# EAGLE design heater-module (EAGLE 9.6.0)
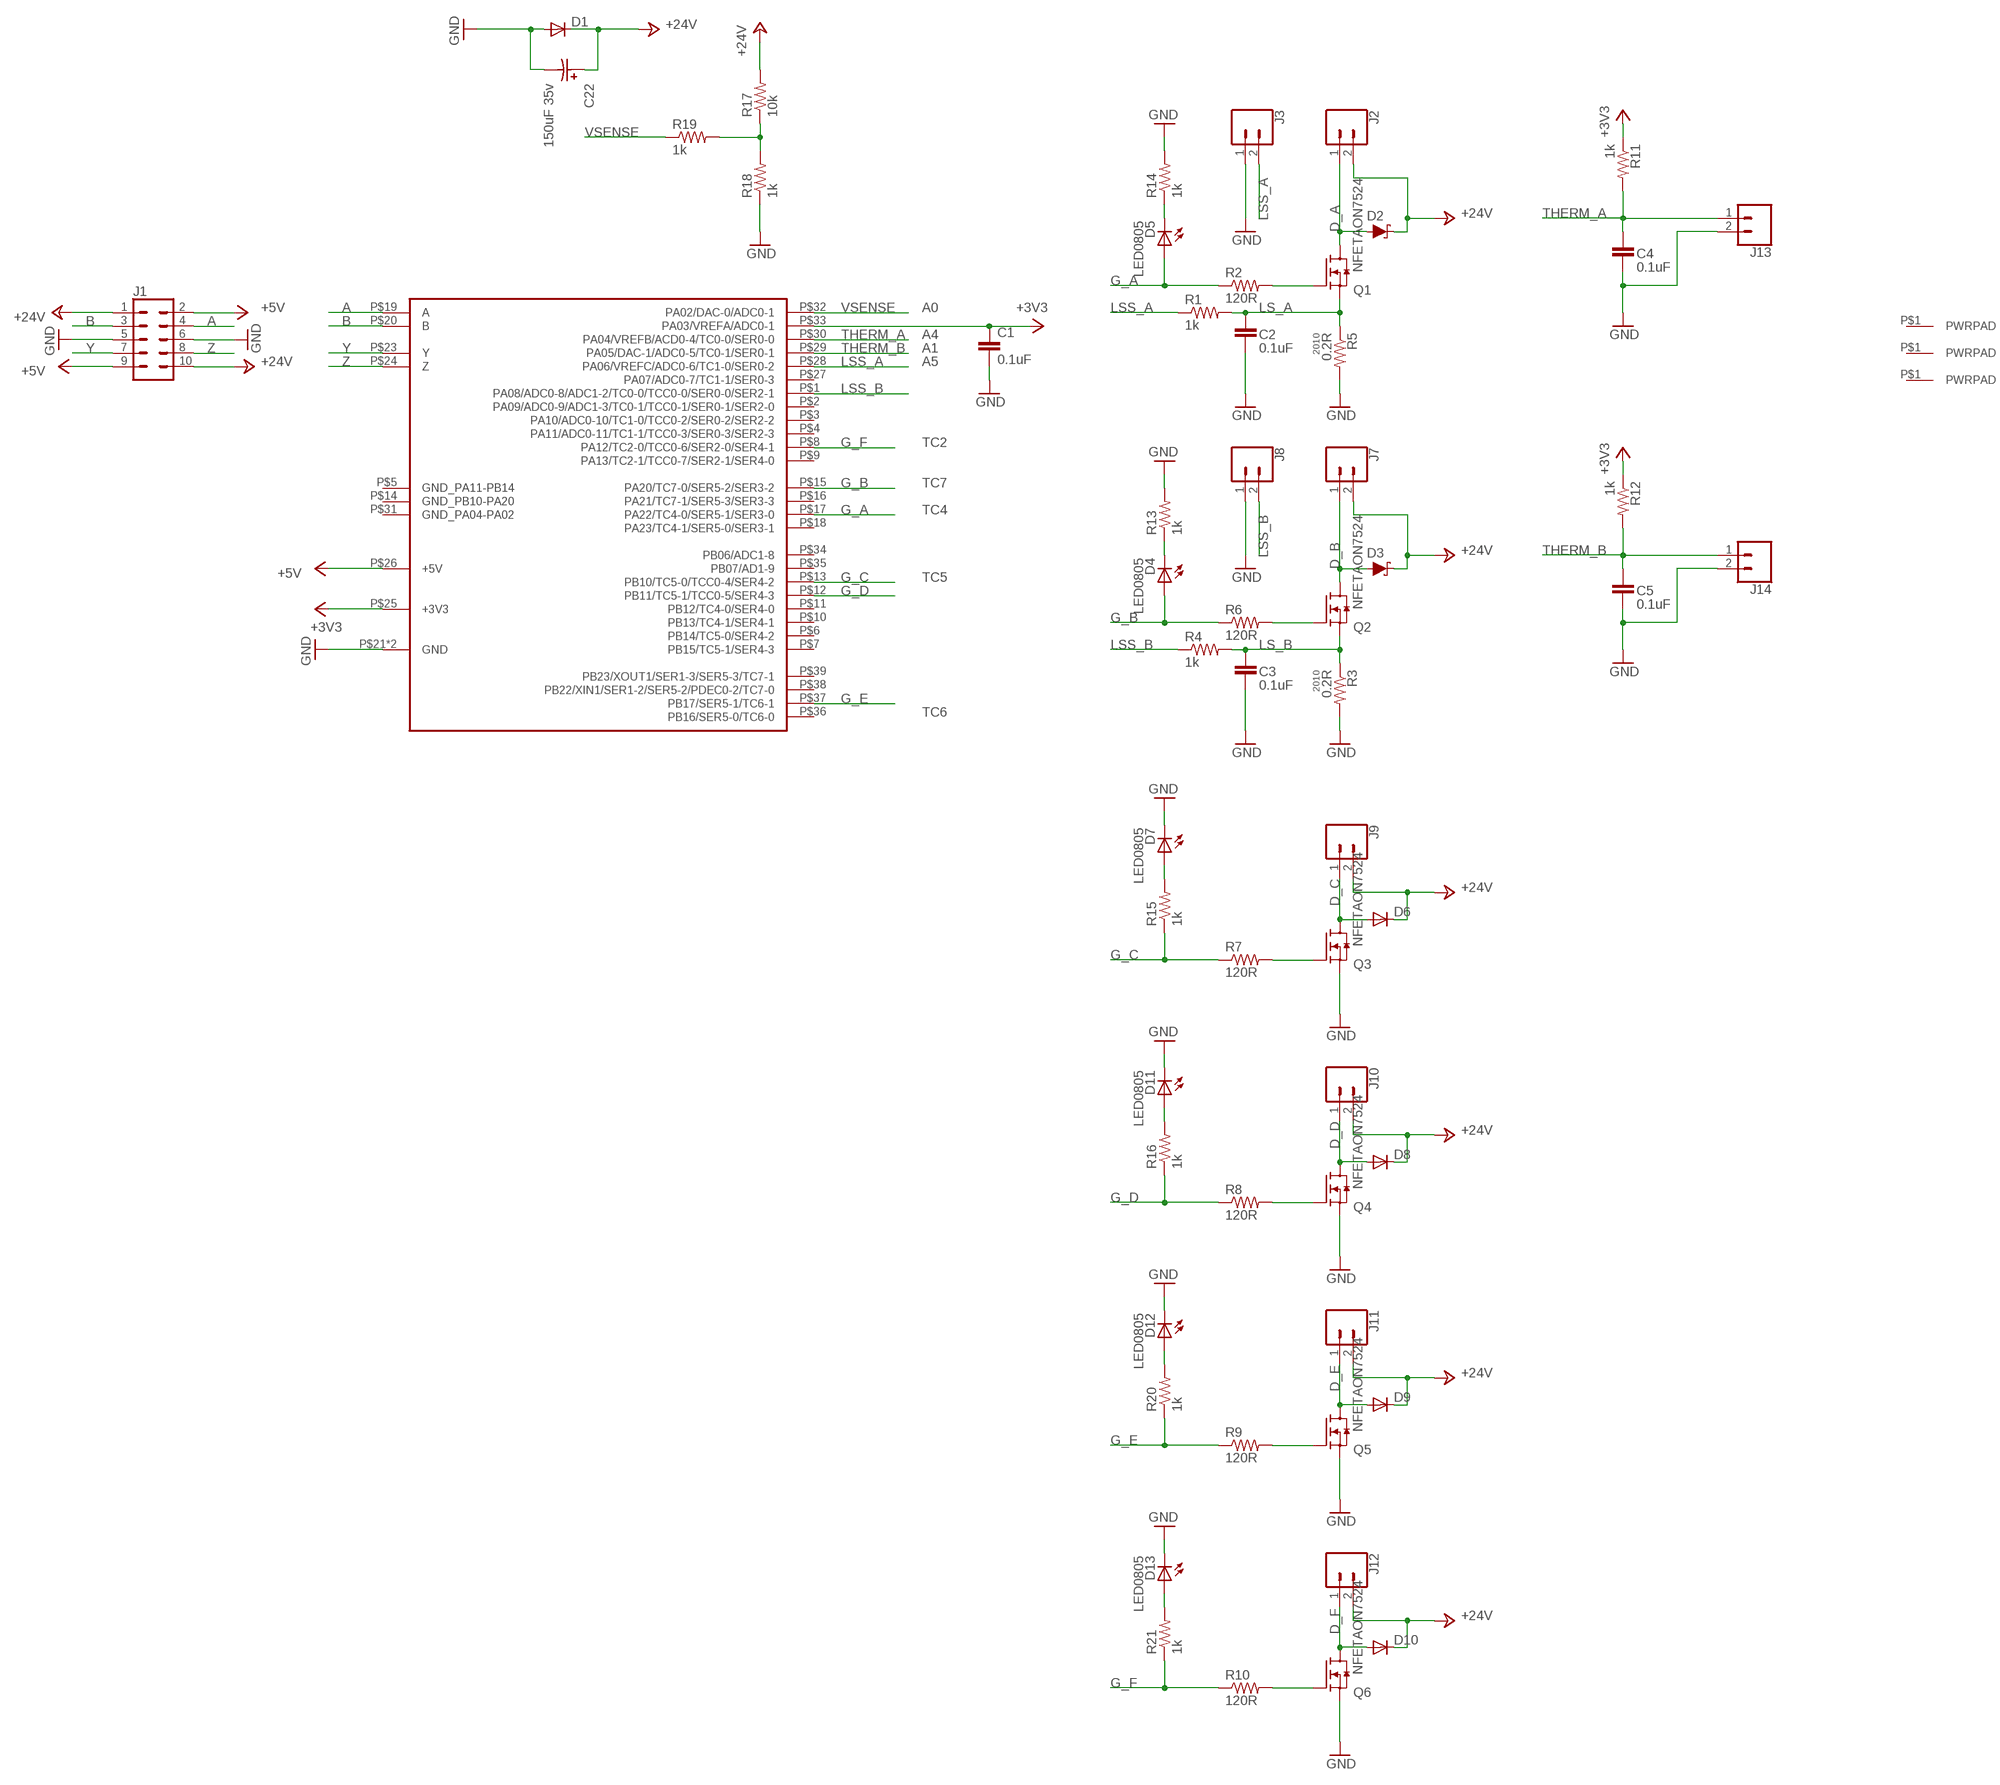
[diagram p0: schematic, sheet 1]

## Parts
C1  0.1uF  CAP0805  [0805]
C2  0.1uF  CAP0805  [0805]
C3  0.1uF  CAP0805  [0805]
C4  0.1uF  CAP0805  [0805]
C5  0.1uF  CAP0805  [0805]
C22  150uF 35v  CAP-POLCAP_POL_SMD6.6X6.6  [SMD-ELEC-CAP]
D1  DIODESMA403D  [SMA-403D]
D2  DIODE-SCHOTTKYPMEG045V100EPDAZ  [DIODE_PMEG045T100EPDZ]
D3  DIODE-SCHOTTKYPMEG045V100EPDAZ  [DIODE_PMEG045T100EPDZ]
D4  LED0805  [LED0805]
D5  LED0805  [LED0805]
D6  DIODESOD123HE  [SOD-123HE]
D7  LED0805  [LED0805]
D8  DIODESOD123HE  [SOD-123HE]
D9  DIODESOD123HE  [SOD-123HE]
D10  DIODESOD123HE  [SOD-123HE]
D11  LED0805  [LED0805]
D12  LED0805  [LED0805]
D13  LED0805  [LED0805]
J1  CONN_05X2SHD_LOCK_LATCH  [2X5-SHROUDED_LOCK_LATCH]
J2  CONN_02LOCK_LONGPADS  [1X02_LOCK_LONGPADS]
J3  CONN_02LOCK  [1X02_LOCK]
J4  PWRPADM3-SKINNY  [PWRPAD_3-25MM-SKINNY]
J5  PWRPADM3-SKINNY  [PWRPAD_3-25MM-SKINNY]
J6  PWRPADM3-SKINNY  [PWRPAD_3-25MM-SKINNY]
J7  CONN_02LOCK_LONGPADS  [1X02_LOCK_LONGPADS]
J8  CONN_02LOCK  [1X02_LOCK]
J9  CONN_02LOCK_LONGPADS  [1X02_LOCK_LONGPADS]
J10  CONN_02LOCK_LONGPADS  [1X02_LOCK_LONGPADS]
J11  CONN_02LOCK_LONGPADS  [1X02_LOCK_LONGPADS]
J12  CONN_02LOCK_LONGPADS  [1X02_LOCK_LONGPADS]
J13  CONN_02LOCK_LONGPADS  [1X02_LOCK_LONGPADS]
J14  CONN_02LOCK_LONGPADS  [1X02_LOCK_LONGPADS]
Q1  NFETAON7524  [TRANS_AON7408]
Q2  NFETAON7524  [TRANS_AON7408]
Q3  NFETAON7524  [TRANS_AON7408]
Q4  NFETAON7524  [TRANS_AON7408]
Q5  NFETAON7524  [TRANS_AON7408]
Q6  NFETAON7524  [TRANS_AON7408]
R1  1k  RESISTOR0805-RES  [0805]
R2  120R  RESISTOR0805-RES  [0805]
R3  0.2R  RESISTOR2010  [R2010]
R4  1k  RESISTOR0805-RES  [0805]
R5  0.2R  RESISTOR2010  [R2010]
R6  120R  RESISTOR0805-RES  [0805]
R7  120R  RESISTOR0805-RES  [0805]
R8  120R  RESISTOR0805-RES  [0805]
R9  120R  RESISTOR0805-RES  [0805]
R10  120R  RESISTOR0805-RES  [0805]
R11  1k  RESISTOR0805-RES  [0805]
R12  1k  RESISTOR0805-RES  [0805]
R13  1k  RESISTOR0805-RES  [0805]
R14  1k  RESISTOR0805-RES  [0805]
R15  1k  RESISTOR0805-RES  [0805]
R16  1k  RESISTOR0805-RES  [0805]
R17  10k  RESISTOR0805-RES  [0805]
R18  1k  RESISTOR0805-RES  [0805]
R19  1k  RESISTOR0805-RES  [0805]
R20  1k  RESISTOR0805-RES  [0805]
R21  1k  RESISTOR0805-RES  [0805]
U1  UCBUS_MODULE_EXT  [UCBUS_MODULE_EXT]

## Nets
+3V3: C1.1 R11.1 R12.1 U1.P$25(+3V3) U1.P$33(PA03/VREFA/ADC0-1)
+5V: J1.2 J1.9 U1.P$26(+5V)
+24V: C22.A D1.P$1(C) D2.3(C) D3.3(C) D6.P$1(C) D8.P$1(C) D9.P$1(C) D10.P$1(C) J1.1 J1.10 J2.2 J7.2 J9.2 J10.2 J11.2 J12.2 R17.2
A: J1.4 U1.P$19(A)
B: J1.3 U1.P$20(B)
D_A: D2.1(A) D2.2(A) J2.1 Q1.9(D)
D_B: D3.1(A) D3.2(A) J7.1 Q2.9(D)
D_C: D6.P$2(A) J9.1 Q3.9(D)
D_D: D8.P$2(A) J10.1 Q4.9(D)
D_E: D9.P$2(A) J11.1 Q5.9(D)
D_F: D10.P$2(A) J12.1 Q6.9(D)
G_A: D5.1(A) R2.1 U1.P$17(PA22/TC4-0/SER5-1/SER3-0)
G_B: D4.1(A) R6.1 U1.P$15(PA20/TC7-0/SER5-2/SER3-2)
G_C: R7.1 R15.1 U1.P$13(PB10/TC5-0/TCC0-4/SER4-2)
G_D: R8.1 R16.1 U1.P$12(PB11/TC5-1/TCC0-5/SER4-3)
G_E: R9.1 R20.1 U1.P$37(PB17/SER5-1/TC6-1)
G_F: R10.1 R21.1 U1.P$8(PA12/TC2-0/TCC0-6/SER2-0/SER4-1)
GND: C1.2 C2.2 C3.2 C4.2 C5.2 C22.C D1.P$2(A) D7.2(C) D11.2(C) D12.2(C) D13.2(C) J1.5 J1.6 J3.1 J8.1 J13.2 J14.2 Q3.1(S) Q3.2(S) Q3.3(S) Q4.1(S) Q4.2(S) Q4.3(S) Q5.1(S) Q5.2(S) Q5.3(S) Q6.1(S) Q6.2(S) Q6.3(S) R3.2 R5.2 R13.2 R14.2 R18.1 U1.P$21(GND) U1.P$22(GND)
LS_A: C2.1 Q1.1(S) Q1.2(S) Q1.3(S) R1.2 R5.1
LS_B: C3.1 Q2.1(S) Q2.2(S) Q2.3(S) R3.1 R4.2
LSS_A: J3.2 R1.1 U1.P$28(PA06/VREFC/ADC0-6/TC1-0/SER0-2)
LSS_B: J8.2 R4.1 U1.P$1(PA08/ADC0-8/ADC1-2/TC0-0/TCC0-0/SER0-0/SER2-1)
N$1: Q1.4(G) R2.2
N$2: Q2.4(G) R6.2
N$3: Q3.4(G) R7.2
N$4: Q4.4(G) R8.2
N$5: Q5.4(G) R9.2
N$6: Q6.4(G) R10.2
N$7: D4.2(C) R13.1
N$8: D5.2(C) R14.1
N$9: D7.1(A) R15.2
N$10: D11.1(A) R16.2
N$11: D12.1(A) R20.2
N$12: D13.1(A) R21.2
N$17: R17.1 R18.2 R19.2
THERM_A: C4.1 J13.1 R11.2 U1.P$30(PA04/VREFB/ACD0-4/TC0-0/SER0-0)
THERM_B: C5.1 J14.1 R12.2 U1.P$29(PA05/DAC-1/ADC0-5/TC0-1/SER0-1)
VSENSE: R19.1 U1.P$32(PA02/DAC-0/ADC0-1)
Y: J1.7 U1.P$23(Y)
Z: J1.8 U1.P$24(Z)
Unconnected: J4.P$1(PWRPAD) J5.P$1(PWRPAD) J6.P$1(PWRPAD) U1.P$2(PA09/ADC0-9/ADC1-3/TC0-1/TCC0-1/SER0-1/SER2-0) U1.P$3(PA10/ADC0-10/TC1-0/TCC0-2/SER0-2/SER2-2) U1.P$4(PA11/ADC0-11/TC1-1/TCC0-3/SER0-3/SER2-3) U1.P$5(GND_PA11-PB14) U1.P$6(PB14/TC5-0/SER4-2) U1.P$7(PB15/TC5-1/SER4-3) U1.P$9(PA13/TC2-1/TCC0-7/SER2-1/SER4-0) U1.P$10(PB13/TC4-1/SER4-1) U1.P$11(PB12/TC4-0/SER4-0) U1.P$14(GND_PB10-PA20) U1.P$16(PA21/TC7-1/SER5-3/SER3-3) U1.P$18(PA23/TC4-1/SER5-0/SER3-1) U1.P$27(PA07/ADC0-7/TC1-1/SER0-3) U1.P$31(GND_PA04-PA02) U1.P$34(PB06/ADC1-8) U1.P$35(PB07/AD1-9) U1.P$36(PB16/SER5-0/TC6-0) U1.P$38(PB22/XIN1/SER1-2/SER5-2/PDEC0-2/TC7-0) U1.P$39(PB23/XOUT1/SER1-3/SER5-3/TC7-1)

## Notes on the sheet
- A0
- A4
- A1
- A5
- TC2
- TC7
- TC4
- TC5
- TC6

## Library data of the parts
C1-C5 = passives:CAP: Capacitor; PACKAGE: 0805
C22 = passives:CAP-POL
D1 D6 D8-D10 = passives:DIODE: DIODE
D2 D3 = power:DIODE-SCHOTTKY: Schottky diode
D4 D5 D7 D11-D13 = lights:LED: LED
J1 = SparkFun-Connectors:CONN_05X2: Multi connection point. Often used as Generic Header-pin footprint for 0.1 inch spaced/style header connections For AVR SPI programming port, see special device with nice symbol: "AVR_SPI_PROG_5x2.dev" You can populate with any combo of single row headers, but if you'd like an exact match, check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
J2 J3 J7-J14 = SparkFun-Connectors:CONN_02: Multi connection point. Often used as Generic Header-pin footprint for 0.1 inch spaced/style header connections
J4-J6 = connector:PWRPAD
Q1-Q6 = power:NFET
R1 R2 R4 R6-R21 = passives:RESISTOR: Resistor; PACKAGE: 0805
R3 R5 = passives:RESISTOR: Resistor; PACKAGE: 2010
U1 = connector:UCBUS_MODULE_EXT

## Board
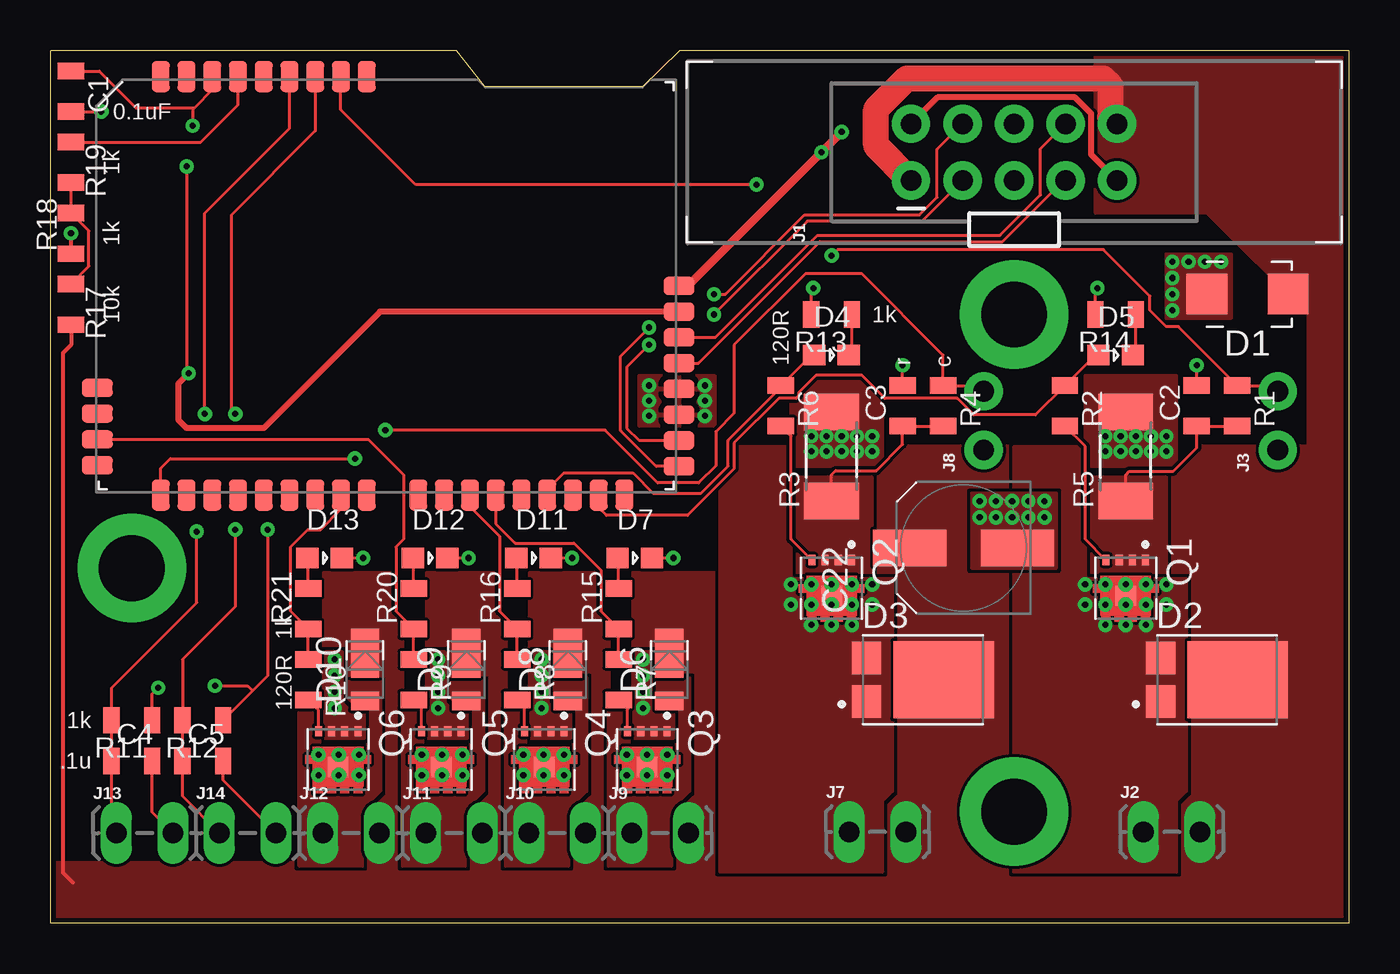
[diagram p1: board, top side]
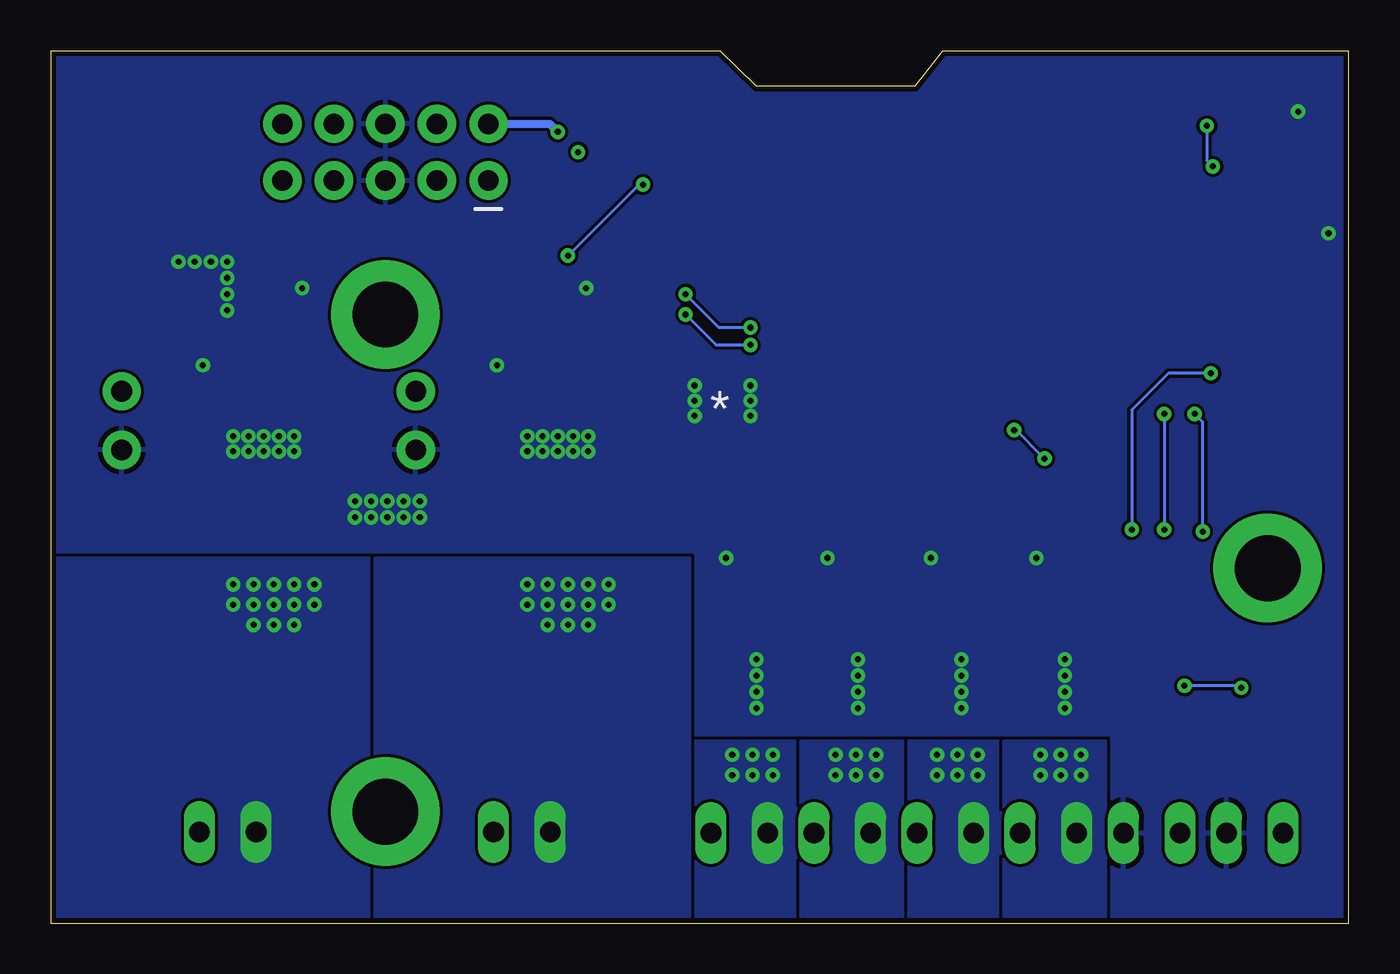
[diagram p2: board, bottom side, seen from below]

Size 64 x 43 mm. Coordinates in mm from the lower left corner, seen from the top.
Outline: 64,43 31,43 29.2,41.25 21.4,41.25 20,43 0,43 0,0 64,0 64,43
Copper layers (1*16): Top 0.035mm / dielectric 1.5mm / Bottom 0.035mm
Design rules "default *": minimum track width 6mil, minimum drill 10mil, track to track 6mil, track to pad 6mil, pad to pad 6mil, via to via 6mil, smd to smd 0mil, copper to edge 10mil, drill to drill 6mil, minimum pad ring 10mil, minimum via ring 8mil, stop-mask expansion 4mil, vias tented up to drill 35mil, thermal gap 10mil

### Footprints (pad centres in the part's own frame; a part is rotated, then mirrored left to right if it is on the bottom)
0805 = smd 0.8 x 1.3: 1 -1,0; 2 1,0
SMD-ELEC-CAP = smd 1.8 x 3.6: A 0,2.65; C 0,-2.65
SMA-403D = smd 2 x 2: P$1 -2,0; P$2 2,0
DIODE_PMEG045T100EPDZ = smd 1.44 x 1.6: 1 -2.78,-1.065; 2 -2.78,1.065 | smd 4.96 x 3.8: 3 1.02,0
LED0805 = smd 1.1 x 1: 1 -0.85,0; 2 0.85,0
SOD-123HE = smd 2.4 x 1.4: P$1 0.8,0 | smd 0.9 x 1.4: P$2 -1.55,0
2X5-SHROUDED_LOCK_LATCH = drill 1.016 pad 1.88: 1 -1.397,5.08; 2 1.397,5.08; 3 -1.397,2.54; 4 1.397,2.54; 5 -1.397,0; 6 1.397,0; 7 -1.397,-2.54; 8 1.397,-2.54; 9 -1.397,-5.08; 10 1.397,-5.08
1X02_LOCK_LONGPADS = drill 1.016 long: 1 -0.127,0; 2 2.667,0
1X02_LOCK = drill 1.016 pad 1.88: 1 -0.178,0; 2 2.718,0
PWRPAD_3-25MM-SKINNY = drill 3.25 pad 5.35: P$1 0,0
TRANS_AON7408 = smd 0.5 x 0.35: 1 -1.4,0.975; 2 -1.4,0.325; 3 -1.4,-0.325; 4 -1.4,-0.975 | smd 1 x 1: 9 0.36,0
R2010 = smd 1.8 x 2.7: 1 -2.2,0; 2 2.2,0
UCBUS_MODULE_EXT = smd 0.889 x 1.524: P$1 3.175,-0.152; P$2 4.445,-0.152; P$3 5.715,-0.152; P$4 6.985,-0.152; P$5 8.255,-0.152; P$6 9.525,-0.152; P$7 10.795,-0.152; P$8 12.065,-0.152; P$9 13.335,-0.152; P$10 15.875,-0.152; P$11 17.145,-0.152; P$12 18.415,-0.152; P$13 19.685,-0.152; P$14 20.955,-0.152; P$15 22.225,-0.152; P$16 23.495,-0.152; P$17 24.765,-0.152; P$18 26.035,-0.152; P$27 13.335,20.472; P$28 12.065,20.472; P$29 10.795,20.472; P$30 9.525,20.472; P$31 8.255,20.472; P$32 6.985,20.472; P$33 5.715,20.472; P$34 4.445,20.472; P$35 3.175,20.472 | smd 1.524 x 0.889: P$19 28.727,1.27; P$20 28.727,2.54; P$21 28.727,3.81; P$22 28.727,5.08; P$23 28.727,6.35; P$24 28.727,7.62; P$25 28.727,8.89; P$26 28.727,10.16; P$36 0.05,1.32; P$37 0.05,2.59; P$38 0.05,3.86; P$39 0.05,5.13

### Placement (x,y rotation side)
C1  1,41 270 top
C2  56.5,25.5 90 top
C3  42,25.5 90 top
C4  4,8 0 top
C5  7.5,8 0 top
C22  45,18.5 90 top
D1  59,31 180 top
D2  57.5,12 0 top
D3  43,12 0 top
D4  38.5,28 0 top
D5  52.5,28 0 top
D6  30.5,12.5 90 top
D7  28.8,18 0 top
D8  25.5,12.5 90 top
D9  20.5,12.5 90 top
D10  15.5,12.5 90 top
D11  23.8,18 0 top
D12  18.7,18 0 top
D13  13.5,18 0 top
J1  47.5,38 90 top
J2  54,4.5 0 top
J3  60.5,23.5 90 top
J4  47.5,5.5 0 top
J5  47.5,30 0 top
J6  4,17.5 0 top
J7  39.5,4.5 0 top
J8  46,23.5 90 top
J9  28.78,4.45 0 top
J10  23.7,4.45 0 top
J11  18.62,4.45 0 top
J12  13.54,4.45 0 top
J13  3.36,4.45 0 top
J14  8.44,4.45 0 top
Q1  53,16.5 270 top
Q2  38.5,16.5 270 top
Q3  29.41,8.06 270 top
Q4  24.34,8.06 270 top
Q5  19.25,8.06 270 top
Q6  14.18,8.06 270 top
R1  58.5,25.5 270 top
R2  50,25.5 270 top
R3  38.5,23 90 top
R4  44,25.5 270 top
R5  53,23 90 top
R6  36,25.5 270 top
R7  28,12 270 top
R8  23,12 270 top
R9  17.9,12 270 top
R10  12.7,12 270 top
R11  4,10 180 top
R12  7.5,10 180 top
R13  38.5,30 180 top
R14  52.5,30 180 top
R15  28,15.5 90 top
R16  23,15.5 90 top
R17  1,30.5 270 top
R18  1,34 90 top
R19  1,37.5 270 top
R20  17.9,15.5 90 top
R21  12.7,15.5 90 top
U1  2.25,21.25 0 top

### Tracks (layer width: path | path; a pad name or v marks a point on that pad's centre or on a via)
+3V3  (via drill 0.3)
  Top 0.152: C1.1 2.4,42 4.2,40.2 7.1,40.2 | 7.1,40.2 7.96,41.06 U1.P$33 | 7.1,40.2 7,40.1 v7,39.3 | v6.8,27.1 6.7,27.2 v6.7,37.3 | v10.7,19.4 10.7,12.2 9.95,11.45 | 9.95,11.45 R12.1 | R11.1 5,11.3 v5.3,11.6 | v8.1,11.7 9.7,11.7 9.95,11.45
  Top 0.305: U1.P$25 16.24,30.14 10.5,24.4 6.7,24.4 6.3,24.8 6.3,26.6 v6.8,27.1
  Bottom 0.152: v7,39.3 7,37.6 v6.7,37.3 | v6.8,27.1 8.9,27.1 10.7,25.3 v10.7,19.4 | v5.3,11.6 5.4,11.7 v8.1,11.7
+5V  (via drill 0.3)
  Top 0.305: J1.9 51.3,37.88 51.3,39.9 50.5,40.7 43.72,40.7 J1.2
  Top 0.406: U1.P$26 31.41,31.41 v38,38 v39,39
  Bottom 0.406: J1.2 39.4,39.4 v39,39
+24V
  Top 0.203: R17.2 1,28.5 0.6,28.1 0.6,2.5 1.1,2
  Top 1.27: J1.1 40.69,38.33 40.69,40.11 42.22,41.64 51.89,41.64 52.24,41.29 52.24,39.74 J1.10
  pour Top (rank 4, no thermals): 55,23.5 55,2.5 62,2.5 62,23.5
  pour Top (rank 4, no thermals): 40.5,23.5 40.5,2.5 47.5,2.5 47.5,23.5
  pour Top (rank 3, no thermals): 29.6,12.1 29.6,13.4 28.7,13.4 28.7,17.3 33,17.3 33,0.9 30.6,0.9 30.6,5.6 31.5,6.5 31.5,12.1
  pour Top (rank 3, no thermals): 24.52,12.1 24.52,13.4 23.62,13.4 23.62,17.3 27.52,17.3 27.52,0.9 25.52,0.9 25.52,5.6 26.42,6.5 26.42,12.1
  pour Top (rank 3, no thermals): 19.44,12.1 19.44,13.4 18.54,13.4 18.54,17.3 22.44,17.3 22.44,0.9 20.44,0.9 20.44,5.6 21.34,6.5 21.34,12.1
  pour Top (rank 3, no thermals): 14.36,12.1 14.36,13.4 13.46,13.4 13.46,17.3 17.36,17.3 17.36,0.9 15.36,0.9 15.36,5.6 16.26,6.5 16.26,12.1
  pour Top (rank 3, no thermals): 51.5,35 51.5,45 66,45 66,-2 -2,-2 -2,3 62,3 62,30 57,35
A  (via drill 0.3)
  Top 0.152: U1.P$19 29.85,22.52 28.09,24.27 28.09,27.95 v29.5,29.36 | v32.7,31 33.27,31 37.17,34.91 42.83,34.91 43.7,35.77 43.7,38.14 J1.4
  Bottom 0.152: v29.5,29.36 31.06,29.36 v32.7,31
B  (via drill 0.3)
  Top 0.152: J1.3 42.96,34.6 37.3,34.6 v32.7,30 | v29.5,28.5 28.4,27.4 28.4,24.4 29.01,23.79 U1.P$20
  Bottom 0.152: v32.7,30 31.2,28.5 v29.5,28.5
D_A  (via drill 0.3)
  other vias: 53,15.7 53,16.7 54,16.7 52,16.7 52,15.7 54,15.7 55,15.7 54,14.7 53,14.7 52,14.7 51,15.7 51,16.7 55,16.7
  pour Top (rank 2, no thermals): 56,17 56,6.5 55.5,6 55.5,2.5 47.5,2.5 47.5,23.5 51,23.5 51,17
  pour Bottom (rank 2, no thermals): 48,18 48,-0.5 64.5,-0.5 64.5,18
D_B  (via drill 0.3)
  other vias: 38.5,15.7 38.5,16.7 39.5,16.7 37.5,16.7 37.5,15.7 39.5,15.7 40.5,15.7 39.5,14.7 38.5,14.7 37.5,14.7 36.5,15.7 36.5,16.7 40.5,16.7
  pour Top (rank 2, no thermals): 41.5,17 41.5,6.5 41,6 41,2.5 33,2.5 33,23.5 36.5,23.5 36.5,17
  pour Bottom (no thermals): 32.5,18 32.5,-0.5 48,-0.5 48,18
D_C  (via drill 0.3)
  other vias: 29.4,7.3 29.4,8.3 30.4,8.3 28.4,8.3 28.4,7.3 30.4,7.3
  pour Top (rank 2, no thermals): 29.6,12.1 31.5,12.1 31.5,6.5 30.6,5.6 30.6,2.8 27.9,2.8 27.5,2.8 27.5,10.6 28.7,10.6 28.7,9.1 30.7,9.1 30.7,10.5 30,10.5 29.6,10.9
  pour Bottom (rank 2, no thermals): 32.5,9 27,9 27,-0.5 32.5,-0.5
D_D  (via drill 0.3)
  other vias: 24.3,7.3 24.3,8.3 25.3,8.3 23.3,8.3 23.3,7.3 25.3,7.3
  pour Top (rank 2, no thermals): 24.52,12.1 26.42,12.1 26.42,6.5 25.52,5.6 25.52,2.8 22.82,2.8 22.42,2.8 22.42,10.6 23.62,10.6 23.62,9.1 25.62,9.1 25.62,10.5 24.92,10.5 24.52,10.9
  pour Bottom (no thermals): 27,9 22,9 22,-0.5 27,-0.5
D_E  (via drill 0.3)
  other vias: 19.3,7.3 19.3,8.3 20.3,8.3 18.3,8.3 18.3,7.3 20.3,7.3
  pour Top (rank 2, no thermals): 19.44,12.1 21.34,12.1 21.34,6.5 20.44,5.6 20.44,2.8 17.74,2.8 17.34,2.8 17.34,10.6 18.54,10.6 18.54,9.1 20.54,9.1 20.54,10.5 19.84,10.5 19.44,10.9
  pour Bottom (rank 2, no thermals): 22,9 17,9 17,-0.5 22,-0.5
D_F  (via drill 0.3)
  other vias: 14.2,7.3 14.2,8.3 15.2,8.3 13.2,8.3 13.2,7.3 15.2,7.3
  pour Top (rank 2, no thermals): 14.36,12.1 16.26,12.1 16.26,6.5 15.36,5.6 15.36,2.8 12.26,2.8 12.26,10.6 13.46,10.6 13.46,9.1 15.46,9.1 15.46,10.5 14.76,10.5 14.36,10.9
  pour Bottom (no thermals): 17,9 12,9 12,-0.5 17,-0.5
G_A
  Top 0.152: D5.1 51.5,28 R2.1 48.55,25.05 45.52,25.05 44.69,25.87 41.13,25.87 40,27 37.73,27 36.88,26.15 36.88,26 36.74,25.87 35.9,25.87 33.7,23.67 33.7,22.4 31.4,20.1 27.4,20.1 27.02,20.48 U1.P$17
G_B
  Top 0.152: D4.1 37.5,28 R6.1 36,26.4 33.4,23.8 33.4,22.53 32.07,21.2 29.7,21.2 28.7,22.2 25.3,22.2 24.48,21.38 U1.P$15
G_C
  Top 0.152: R7.1 R15.1 27.12,15.38 27.12,17.4 25.79,18.73 22.9,18.73 21.93,19.69 U1.P$13
G_D
  Top 0.152: R8.1 R16.1 22.12,15.38 22.12,19.08 20.66,20.53 U1.P$12
G_E
  Top 0.152: R9.1 R20.1 17.02,15.38 17.02,18.55 17.4,18.92 17.4,22.1 15.66,23.84 U1.P$37
G_F
  Top 0.152: R10.1 R21.1 11.82,15.38 11.82,18.55 12.68,19.4 13.3,19.4 14.31,20.41 U1.P$8
GND  (via drill 0.3)
  Top 0.152: C3.2 v42,27.5 | C2.2 v56.5,27.5 | D13.2 v15.4,18 | D12.2 v20.6,18 | D11.2 v25.7,18 | D7.2 v30.7,18 | R13.2 37.5,31.2 v37.6,31.3 | R14.2 51.5,31.2 v51.6,31.3 | C1.2 v2.5,40 | J13.2 5,5.47 C4.2 | J14.2 8.5,7.05 C5.2
  Top 0.203: R18.1 v1,34
  other vias: 55,23.25 54.25,23.25 53.5,23.25 52.75,23.25 52,23.25 55,24 54.25,24 53.5,24 52.75,24 52,24 29.5,26.5 29.5,25.75 29.5,25 32.25,26.5 32.25,25.75 32.25,25 40.5,23.25 39.75,23.25 39,23.25 38.25,23.25 37.5,23.25 40.5,24 39.75,24 39,24 38.25,24 37.5,24 29.2,10.6 29.2,11.4 29.2,12.2 29.2,13 24.2,10.6 24.2,11.4 24.2,12.2 24.2,13 19.1,10.6 19.1,11.4 19.1,12.2 19.1,13 14,10.6 14,11.4 14,12.2 14,13 49,20 48.2,20 47.4,20 46.6,20 45.8,20 45.8,20.8 46.6,20.8 47.4,20.8 48.2,20.8 49,20.8 57.7,32.6 56.9,32.6 56.1,32.6 55.3,32.6 55.3,31.8 55.3,31 55.3,30.2
  pour Top (no thermals): 55.5,27 55.5,22.5 51,22.5 51,27
  pour Top: 29,27 32.75,27 32.75,24.5 29,24.5
  pour Top (no thermals): 41,27 41,22.5 36.5,22.5 36.5,27
  pour Bottom (rank 4): -1,44 65,44 65,-1 -1,-1
  pour Top (no thermals): 28.8,13.4 29.6,13.4 29.6,10.9 30,10.5 30.7,10.5 30.7,9.1 28.7,9.1 28.7,13.3
  pour Top (no thermals): 23.72,13.4 24.52,13.4 24.52,10.9 24.92,10.5 25.62,10.5 25.62,9.1 23.62,9.1 23.62,13.3
  pour Top (no thermals): 18.64,13.4 19.44,13.4 19.44,10.9 19.84,10.5 20.54,10.5 20.54,9.1 18.54,9.1 18.54,13.3
  pour Top (no thermals): 13.56,13.4 14.36,13.4 14.36,10.9 14.76,10.5 15.46,10.5 15.46,9.1 13.46,9.1 13.46,13.3
  pour Top: 49.6,17.5 49.6,21.2 45.4,21.2 45.4,17.5
  pour Top (no thermals): 58.2,33 58.2,29.8 55,29.8 55,33
LS_A
  Top 0.152: R5.1 53,22.1 53.17,22.27 55.34,22.27 56.5,23.43 C2.1 R1.2
  pour Top (rank 3, no thermals): 51,22 55,22 55,17 51,17
LS_B
  Top 0.152: R3.1 38.5,22.1 38.7,22.3 40.7,22.3 42,23.6 C3.1 R4.2
  pour Top (rank 3, no thermals): 36.5,22 40.5,22 40.5,17 36.5,17
LSS_A  (via drill 0.3)
  Top 0.152: J3.2 60.22,26.5 R1.1 55.6,29.4 55,29.4 54.2,30.2 54.2,30.9 51.9,33.2 38.8,33.2 v38.5,32.9 | v34.8,36.4 18,36.4 14.3,40.1 14.3,41.71 U1.P$28
  Bottom 0.152: v38.5,32.9 35,36.4 v34.8,36.4
LSS_B  (via drill 0.3)
  Top 0.152: J8.2 45.72,26.5 R4.1 44,28 40,32 37.2,32 33.7,28.5 33.7,25.13 32.79,24.22 32.79,22.55 31.94,21.7 29.93,21.7 27.33,24.3 v16.5,24.3 | U1.P$1 5.42,22.43 5.9,22.9 v15,22.9
  Bottom 0.152: v15,22.9 16.4,24.3 v16.5,24.3
N$1
  Top 0.152: Q1.4 51,18.93 51,23.5 R2.2
N$2
  Top 0.152: Q2.4 36.5,18.93 36.5,24 R6.2
N$3
  Top 0.152: Q3.4 28.44,10.56 R7.2
N$4
  Top 0.152: Q4.4 23.36,10.64 R8.2
N$5
  Top 0.152: Q5.4 18.28,10.62 R9.2
N$6
  Top 0.152: Q6.4 13.2,10.5 R10.2
N$7
  Top 0.152: D4.2 39.5,28.15 R13.1
N$8
  Top 0.152: D5.2 53.5,28.15 R14.1
N$9
  Top 0.152: R15.2 28,17.95 D7.1
N$10
  Top 0.152: R16.2 23,17.95 D11.1
N$11
  Top 0.152: R20.2 17.9,17.95 D12.1
N$12
  Top 0.152: R21.2 12.7,17.95 D13.1
N$17
  Top 0.152: R17.1 1.88,32.38 1.88,34.12 R18.2 R19.2
THERM_A  (via drill 0.3)
  Top 0.152: J13.1 3,4.68 C4.1 R11.2 3,11.6 7.2,15.8 v7.2,19.3 | v7.6,25.1 7.6,35 11.78,39.17 U1.P$30
  Bottom 0.152: v7.2,19.3 7.2,24.7 v7.6,25.1
THERM_B  (via drill 0.3)
  Top 0.152: J14.1 6.5,6.26 C5.1 R12.2 6.5,13 9.1,15.6 v9.1,19.4 | U1.P$29 13.04,39.05 8.9,34.9 8.9,25.3 v9.1,25.1
  Bottom 0.152: v9.1,25.1 v9.1,19.4
VSENSE
  Top 0.152: R19.1 7.4,38.5 9.23,40.34 U1.P$32
Y
  Top 0.152: U1.P$23 31.93,27.6 37.93,33.59 46.93,33.59 49.93,36.6 J1.7
Z
  Top 0.152: U1.P$24 32.77,28.87 37.8,33.9 46.8,33.9 48.8,35.9 48.8,38.16 J1.8

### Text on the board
tPlace: 0.1uF | 1k | 1k | 10k | 1k | 120R | r | c | 1k | 1k | 120R | .1u
bPlace: *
